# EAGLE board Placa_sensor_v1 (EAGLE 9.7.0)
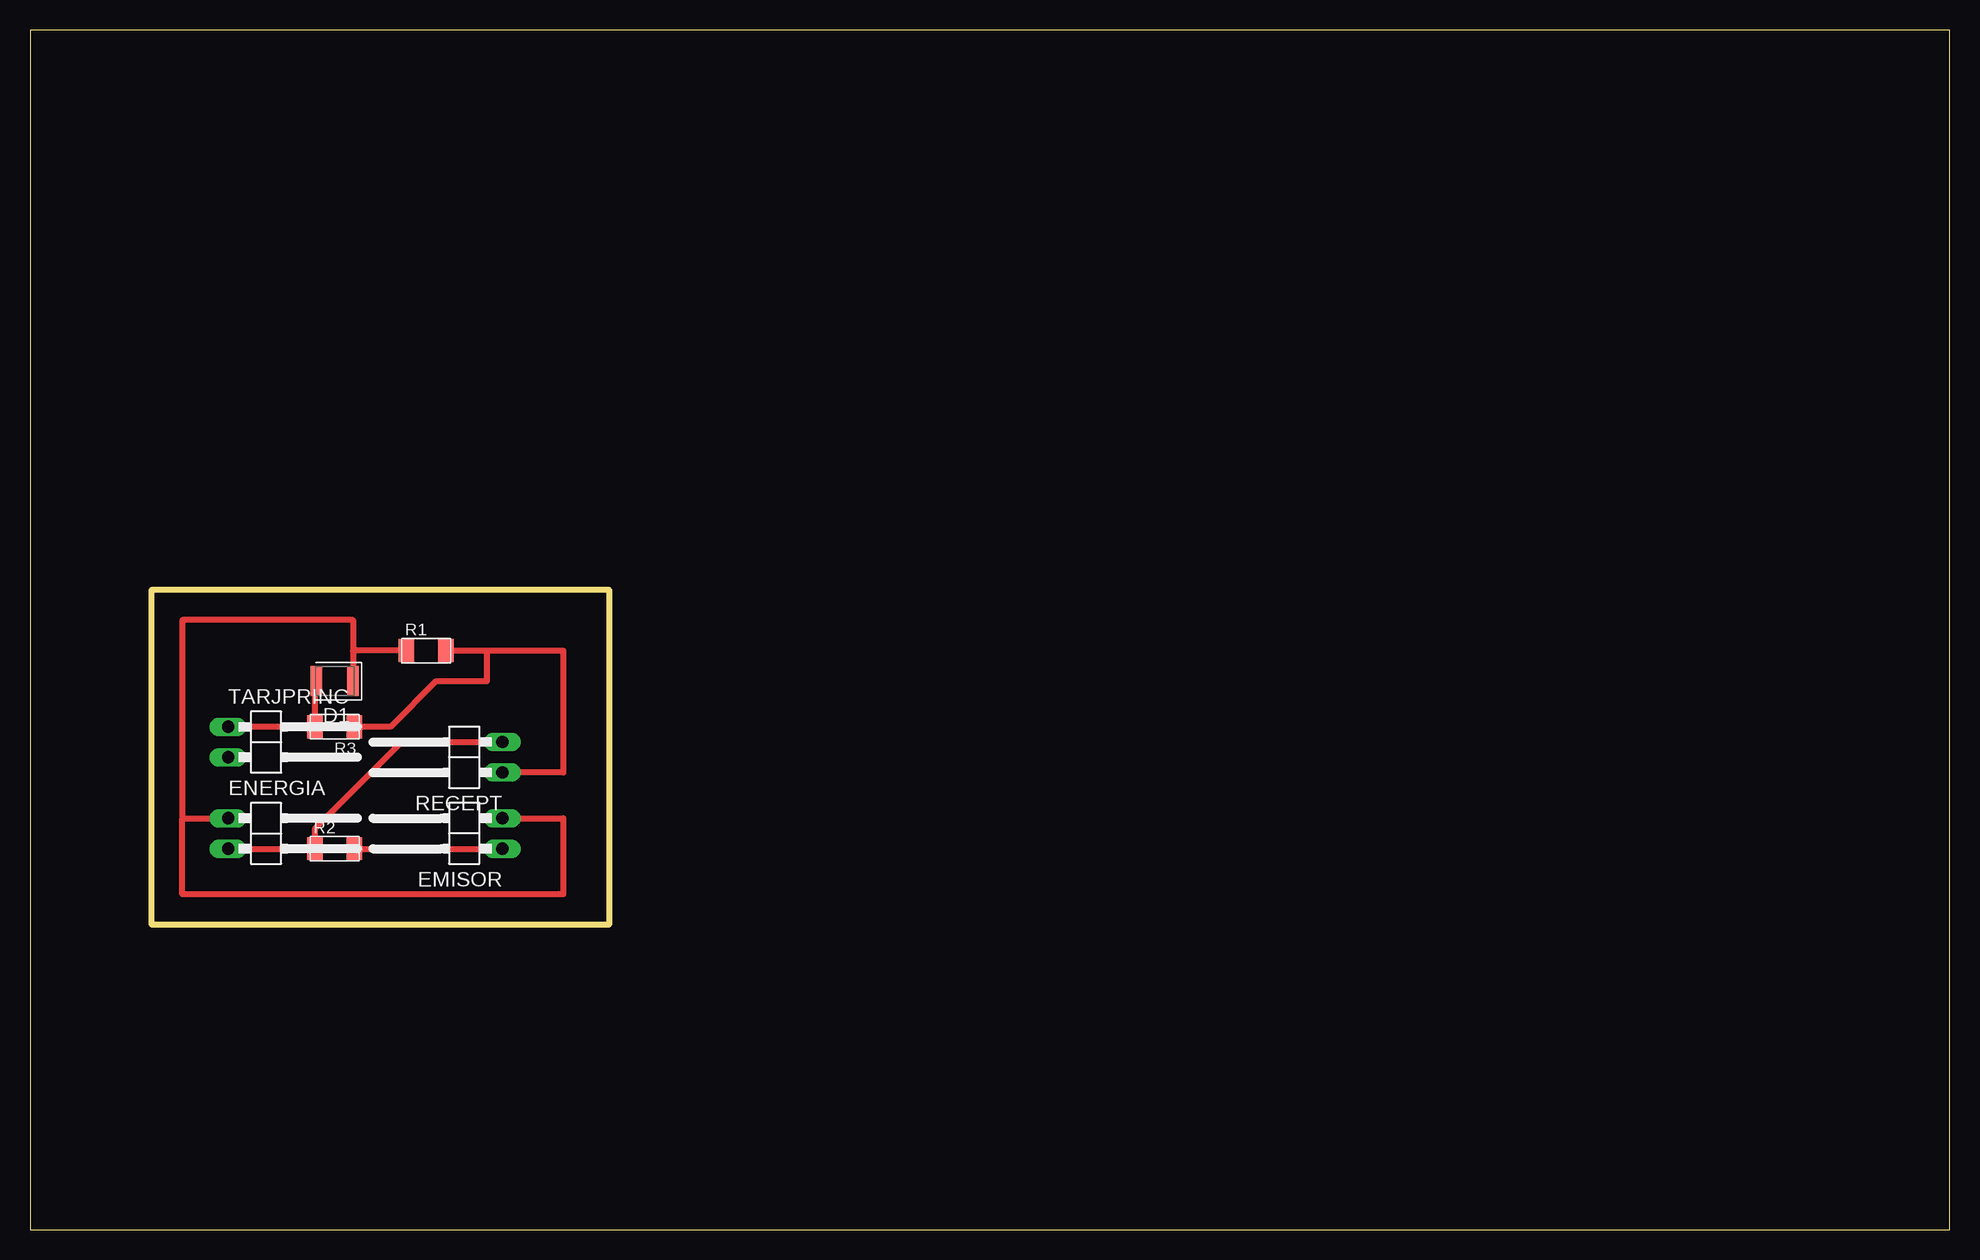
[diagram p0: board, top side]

Size 160 x 100 mm. Coordinates in mm from the lower left corner, seen from the top.
Outline: 0,0 160,0 160,100 0,100 0,0
Outline: 10.16,53.34 48.26,53.34 48.26,25.4 10.16,25.4 10.16,53.34
Copper layers (1*16): Top / Bottom
Stack-up Default Layer Stack: Top User Defined 0.035mm / Dielectric-1 User Defined 1.5mm / Bottom User Defined 0.035mm
Design rules "default": minimum track width 6mil, minimum drill 0.35mm, track to track 6mil, track to pad 6mil, pad to pad 6mil, via to via 6mil, smd to smd 6mil, copper to edge 40mil, drill to drill 6mil, minimum pad ring 10mil, minimum via ring 8mil, stop-mask expansion 4mil, vias tented up to drill 0mil, thermal gap 10mil

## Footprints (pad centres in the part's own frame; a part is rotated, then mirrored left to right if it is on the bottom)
LEDC3224X250N_RND-G = smd 0.962 x 2.512: A 1.525,0; C -1.525,0
1X02/90 = drill 1.016 long: 1 -1.27,-3.81; 2 1.27,-3.81
R1206FAB = smd 1.27 x 1.905: 1 -1.651,0; 2 1.651,0

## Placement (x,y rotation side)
D1  LED_GREEN  [LEDC3224X250N_RND-G]  25.4,45.72 180 top
EMISOR  PINHD-1X2/90  [1X02/90]  35.56,33.02 90 top
ENERGIA  PINHD-1X2/90  [1X02/90]  20.32,33.02 270 top
R1  [R1206FAB]  33.02,48.26 0 top
R2  [R1206FAB]  25.4,31.75 0 top
R3  [R1206FAB]  25.4,41.91 180 top
RECEPT  PINHD-1X2/90  [1X02/90]  35.56,39.37 90 top
TARJPRINC  PINHD-1X2/90  [1X02/90]  20.32,40.64 270 top

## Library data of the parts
D1 = LED; CATEGORY: LED; COLOR: GREEN; DESCRIPTION: CHIP LED ROUND; SUB-CATEGORY: CHIP; TYPE: ROUND_TOP
EMISOR ENERGIA RECEPT TARJPRINC = Connector; CATEGORY: CONNECTOR; SUB-CATEGORY: PIN-HEADER
R1-R3 = fab

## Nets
N$1: ENERGIA.2 R2.1 RECEPT.2
N$2: EMISOR.1 R2.2
N$3: D1.C EMISOR.2 ENERGIA.1 R1.1
N$4: R1.2 R3.1 RECEPT.1
N$5: D1.A R3.2 TARJPRINC.1

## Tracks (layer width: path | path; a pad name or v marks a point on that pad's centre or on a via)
N$1
  Top 0.508: ENERGIA.2 R2.1 23.75,33.4 30.99,40.64 RECEPT.2
N$2
  Top 0.508: R2.2 EMISOR.1
N$3
  Top 0.508: EMISOR.2 44.45,34.29 44.45,27.94 12.7,27.94 12.7,34.29 | 12.7,34.29 ENERGIA.1 | R1.1 26.93,48.26 D1.C 26.93,50.8 12.7,50.8 12.7,34.29
N$4
  Top 0.508: R1.2 38.1,48.26 | 38.1,48.26 44.45,48.26 44.45,38.1 RECEPT.1 | R3.1 30.06,41.91 33.87,45.72 38.1,45.72 38.1,48.26
N$5
  Top 0.508: TARJPRINC.1 R3.2 23.75,45.59 D1.A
